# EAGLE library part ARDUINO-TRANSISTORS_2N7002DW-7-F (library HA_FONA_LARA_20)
MOSFET 2N-CH 60V 0.23A SOT-363
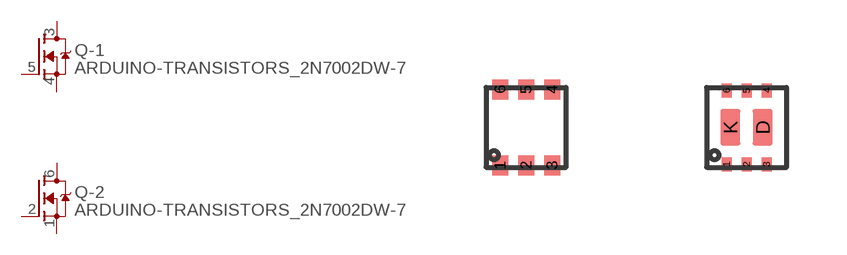
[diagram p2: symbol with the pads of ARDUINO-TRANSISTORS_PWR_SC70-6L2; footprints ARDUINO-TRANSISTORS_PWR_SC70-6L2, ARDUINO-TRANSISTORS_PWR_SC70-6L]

Designator prefix Q; gates -1=ARDUINO-TRANSISTORS_MOSFET_N-CHN -2=ARDUINO-TRANSISTORS_MOSFET_N-CHN

## ARDUINO-TRANSISTORS_2N7002DW-7-FNO_PAD (DATASHEET: http://www.diodes.com/_files/datasheets/ds30120.pdf; DISTRIBUTOR-LINK: http://www.digikey.com/product-detail/en/diodes-incorporated/2N7002DW-7-F/2N7002DW-FDITR-ND/749948; DISTRIBUTOR-PN: 2N7002DW-FDITR-ND; MANUFACTURER: Diodes Incorporated; MANUFACTURER-PN: 2N7002DW-7-F), ARDUINO-TRANSISTORS_2N7002DW-7-FDNPNO_PAD (DATASHEET: DNP; DISTRIBUTOR-LINK: DNP; DISTRIBUTOR-PN: DNP; MANUFACTURER: DNP; MANUFACTURER-PN: DNP)  [ARDUINO-TRANSISTORS_PWR_SC70-6L2]
1  -2:S  pas
2  -2:G  pas
3  -1:D  pas
4  -1:S  pas
5  -1:G  pas
6  -2:D  pas

## ARDUINO-TRANSISTORS_2N7002DW-7-FPAD (DATASHEET: https://www.diodes.com/assets/Datasheets/ds30120.pdf; DISTRIBUTOR-LINK: http://www.digikey.com/product-detail/en/diodes-incorporated/2N7002DW-7-F/2N7002DW-FDICT-ND/750003; DISTRIBUTOR-PN: 2N7002DW-FDICT-ND; MANUFACTURER: Diodes Incorporated; MANUFACTURER-PN: 2N7002DW-7-F; VALUE: 2N7002)  [ARDUINO-TRANSISTORS_PWR_SC70-6L]
1  -1:S  pas
2  -1:G  pas
3  -1:D  pas
4  -2:S  pas
5  -2:G  pas
6  -2:D  pas
D  -1:D  pas
K  -2:D  pas

## Footprint ARDUINO-TRANSISTORS_PWR_SC70-6L2 (pad centres in mm)
smd 0.4 x 0.5: 1 -0.65,-0.95; 2 0,-0.95; 3 0.65,-0.95; 4 0.65,0.95; 5 0,0.95; 6 -0.65,0.95

## Footprint ARDUINO-TRANSISTORS_PWR_SC70-6L (pad centres in mm)
smd 0.25 x 0.35: 1 -0.5,-0.925; 2 0,-0.925; 3 0.5,-0.925; 4 0.5,0.925; 5 0,0.925; 6 -0.5,0.925
smd 0.5 x 0.9: D 0.405,0; K -0.405,0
